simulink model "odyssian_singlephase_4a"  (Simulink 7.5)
settings: Solver=ode23t  StartTime=0.0  StopTime=6  RelTol=1e-6
undefined symbols (not defined in the file or in its folder): dfilt, DiscIntNeverNeededParam
libraries: powerlib x80, powerlib_extras x43, simulink x24, dsparch4 x4
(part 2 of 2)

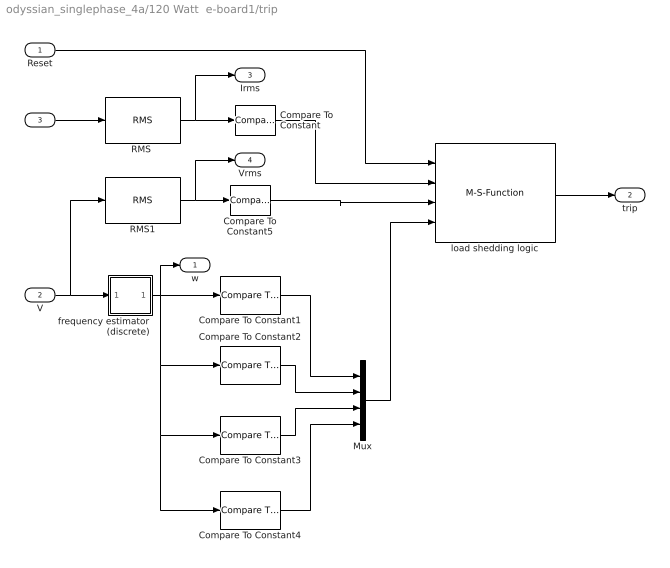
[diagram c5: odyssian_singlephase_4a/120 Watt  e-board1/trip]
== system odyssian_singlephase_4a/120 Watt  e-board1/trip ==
  Reset : Inport
  V : Inport  Port=2
  I : Inport  Port=3
  Compare To Constant : simulink/Logic and Bit Operations/Compare To Constant  SystemSampleTime=-1  relop=>=  const=100  LogicOutDataTypeMode=boolean
  Compare To Constant1 : simulink/Logic and Bit Operations/Compare To Constant  SystemSampleTime=-1  relop=<=  const=59.8  LogicOutDataTypeMode=boolean
  Compare To Constant2 : simulink/Logic and Bit Operations/Compare To Constant  SystemSampleTime=-1  relop=<=  const=59.5  LogicOutDataTypeMode=boolean
  Compare To Constant3 : simulink/Logic and Bit Operations/Compare To Constant  SystemSampleTime=-1  relop=>=  const=60.1  LogicOutDataTypeMode=boolean
  Compare To Constant4 : simulink/Logic and Bit Operations/Compare To Constant  SystemSampleTime=-1  relop=<=  const=58.6  LogicOutDataTypeMode=boolean
  Compare To Constant5 : simulink/Logic and Bit Operations/Compare To Constant  SystemSampleTime=-1  relop=<=  const=100  LogicOutDataTypeMode=boolean
  Mux : Mux
  "RMS " : powerlib_extras/Measurements/RMS  DialogController=POWERSYS.PowerSysDialog  SystemSampleTime=-1  f1=60
  RMS1 : powerlib_extras/Measurements/RMS  DialogController=POWERSYS.PowerSysDialog  SystemSampleTime=-1  f1=60
  frequency estimator (discrete) : Subsystem  mask{dt=0.010}
      mask prompts: dt "sample time"
  load shedding logic : M-S-Function  FunctionName=load_shedding_logic  Parameters=p
  w : Outport  OutDataType=fixdt(1, 16)  OutScaling=2^0
  trip : Outport  Port=2
  Irms : Outport  Port=3  OutDataType=fixdt(1, 16)  OutScaling=2^0
  Vrms : Outport  Port=4  OutDataType=fixdt(1, 16)  OutScaling=2^0
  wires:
  "RMS "/1 -> Compare To Constant/1, Irms/1
  I/1 -> "RMS "/1
  Reset/1 -> load shedding logic/1
  Compare To Constant/1 -> load shedding logic/2
  load shedding logic/1 -> trip/1
  V/1 -> frequency estimator (discrete)/1(v), RMS1/1
  frequency estimator (discrete)/1(w) -> Compare To Constant1/1, w/1, Compare To Constant2/1, Compare To Constant3/1, Compare To Constant4/1
  Compare To Constant1/1 -> Mux/1
  Compare To Constant2/1 -> Mux/2
  Compare To Constant3/1 -> Mux/3
  Compare To Constant4/1 -> Mux/4
  RMS1/1 -> Compare To Constant5/1, Vrms/1
  Compare To Constant5/1 -> load shedding logic/3
  Mux/1 -> load shedding logic/4

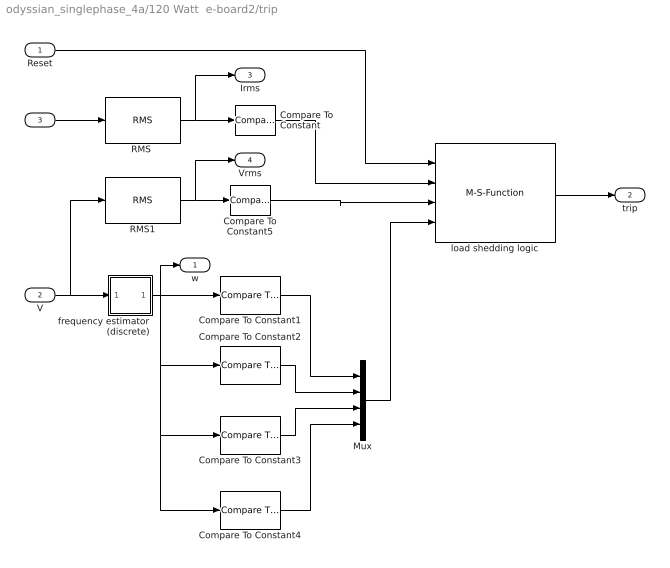
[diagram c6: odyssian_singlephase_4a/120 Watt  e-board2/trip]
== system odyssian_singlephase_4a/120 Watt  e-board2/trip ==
  Reset : Inport
  V : Inport  Port=2
  I : Inport  Port=3
  Compare To Constant : simulink/Logic and Bit Operations/Compare To Constant  SystemSampleTime=-1  relop=>=  const=100  LogicOutDataTypeMode=boolean
  Compare To Constant1 : simulink/Logic and Bit Operations/Compare To Constant  SystemSampleTime=-1  relop=<=  const=59.8  LogicOutDataTypeMode=boolean
  Compare To Constant2 : simulink/Logic and Bit Operations/Compare To Constant  SystemSampleTime=-1  relop=<=  const=59.5  LogicOutDataTypeMode=boolean
  Compare To Constant3 : simulink/Logic and Bit Operations/Compare To Constant  SystemSampleTime=-1  relop=>=  const=60.1  LogicOutDataTypeMode=boolean
  Compare To Constant4 : simulink/Logic and Bit Operations/Compare To Constant  SystemSampleTime=-1  relop=<=  const=58.6  LogicOutDataTypeMode=boolean
  Compare To Constant5 : simulink/Logic and Bit Operations/Compare To Constant  SystemSampleTime=-1  relop=<=  const=100  LogicOutDataTypeMode=boolean
  Mux : Mux
  "RMS " : powerlib_extras/Measurements/RMS  DialogController=POWERSYS.PowerSysDialog  SystemSampleTime=-1  f1=60
  RMS1 : powerlib_extras/Measurements/RMS  DialogController=POWERSYS.PowerSysDialog  SystemSampleTime=-1  f1=60
  frequency estimator (discrete) : Subsystem  mask{dt=0.010}
      mask prompts: dt "sample time"
  load shedding logic : M-S-Function  FunctionName=load_shedding_logic  Parameters=p
  w : Outport  OutDataType=fixdt(1, 16)  OutScaling=2^0
  trip : Outport  Port=2
  Irms : Outport  Port=3  OutDataType=fixdt(1, 16)  OutScaling=2^0
  Vrms : Outport  Port=4  OutDataType=fixdt(1, 16)  OutScaling=2^0
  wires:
  "RMS "/1 -> Compare To Constant/1, Irms/1
  I/1 -> "RMS "/1
  Reset/1 -> load shedding logic/1
  Compare To Constant/1 -> load shedding logic/2
  load shedding logic/1 -> trip/1
  V/1 -> frequency estimator (discrete)/1(v), RMS1/1
  frequency estimator (discrete)/1(w) -> Compare To Constant1/1, w/1, Compare To Constant2/1, Compare To Constant3/1, Compare To Constant4/1
  Compare To Constant1/1 -> Mux/1
  Compare To Constant2/1 -> Mux/2
  Compare To Constant3/1 -> Mux/3
  Compare To Constant4/1 -> Mux/4
  RMS1/1 -> Compare To Constant5/1, Vrms/1
  Compare To Constant5/1 -> load shedding logic/3
  Mux/1 -> load shedding logic/4

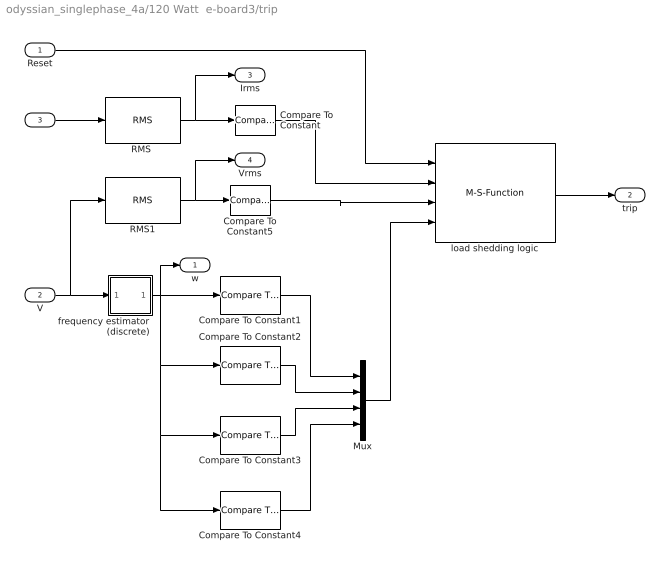
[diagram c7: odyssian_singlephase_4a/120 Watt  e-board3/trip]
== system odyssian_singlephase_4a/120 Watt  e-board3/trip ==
  Reset : Inport
  V : Inport  Port=2
  I : Inport  Port=3
  Compare To Constant : simulink/Logic and Bit Operations/Compare To Constant  SystemSampleTime=-1  relop=>=  const=100  LogicOutDataTypeMode=boolean
  Compare To Constant1 : simulink/Logic and Bit Operations/Compare To Constant  SystemSampleTime=-1  relop=<=  const=59.8  LogicOutDataTypeMode=boolean
  Compare To Constant2 : simulink/Logic and Bit Operations/Compare To Constant  SystemSampleTime=-1  relop=<=  const=59.5  LogicOutDataTypeMode=boolean
  Compare To Constant3 : simulink/Logic and Bit Operations/Compare To Constant  SystemSampleTime=-1  relop=>=  const=60.1  LogicOutDataTypeMode=boolean
  Compare To Constant4 : simulink/Logic and Bit Operations/Compare To Constant  SystemSampleTime=-1  relop=<=  const=58.6  LogicOutDataTypeMode=boolean
  Compare To Constant5 : simulink/Logic and Bit Operations/Compare To Constant  SystemSampleTime=-1  relop=<=  const=100  LogicOutDataTypeMode=boolean
  Mux : Mux
  "RMS " : powerlib_extras/Measurements/RMS  DialogController=POWERSYS.PowerSysDialog  SystemSampleTime=-1  f1=60
  RMS1 : powerlib_extras/Measurements/RMS  DialogController=POWERSYS.PowerSysDialog  SystemSampleTime=-1  f1=60
  frequency estimator (discrete) : Subsystem  mask{dt=0.010}
      mask prompts: dt "sample time"
  load shedding logic : M-S-Function  FunctionName=load_shedding_logic  Parameters=p
  w : Outport  OutDataType=fixdt(1, 16)  OutScaling=2^0
  trip : Outport  Port=2
  Irms : Outport  Port=3  OutDataType=fixdt(1, 16)  OutScaling=2^0
  Vrms : Outport  Port=4  OutDataType=fixdt(1, 16)  OutScaling=2^0
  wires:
  "RMS "/1 -> Compare To Constant/1, Irms/1
  I/1 -> "RMS "/1
  Reset/1 -> load shedding logic/1
  Compare To Constant/1 -> load shedding logic/2
  load shedding logic/1 -> trip/1
  V/1 -> frequency estimator (discrete)/1(v), RMS1/1
  frequency estimator (discrete)/1(w) -> Compare To Constant1/1, w/1, Compare To Constant2/1, Compare To Constant3/1, Compare To Constant4/1
  Compare To Constant1/1 -> Mux/1
  Compare To Constant2/1 -> Mux/2
  Compare To Constant3/1 -> Mux/3
  Compare To Constant4/1 -> Mux/4
  RMS1/1 -> Compare To Constant5/1, Vrms/1
  Compare To Constant5/1 -> load shedding logic/3
  Mux/1 -> load shedding logic/4

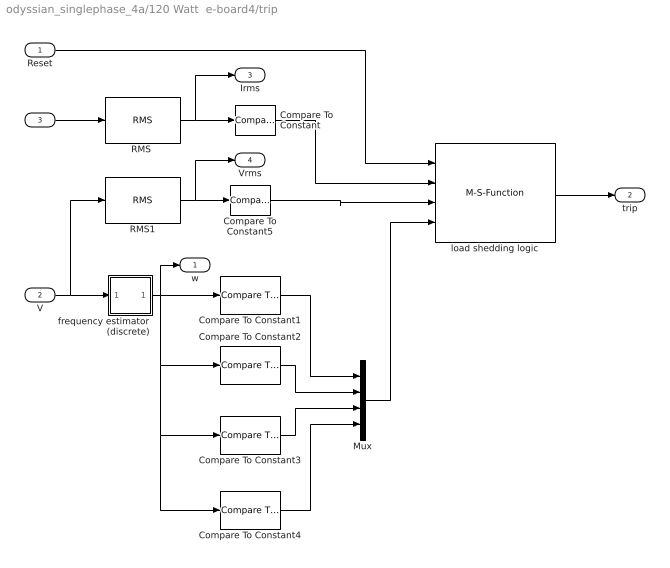
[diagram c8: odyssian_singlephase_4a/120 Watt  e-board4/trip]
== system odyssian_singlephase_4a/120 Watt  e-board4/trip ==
  Reset : Inport
  V : Inport  Port=2
  I : Inport  Port=3
  Compare To Constant : simulink/Logic and Bit Operations/Compare To Constant  SystemSampleTime=-1  relop=>=  const=100  LogicOutDataTypeMode=boolean
  Compare To Constant1 : simulink/Logic and Bit Operations/Compare To Constant  SystemSampleTime=-1  relop=<=  const=59.8  LogicOutDataTypeMode=boolean
  Compare To Constant2 : simulink/Logic and Bit Operations/Compare To Constant  SystemSampleTime=-1  relop=<=  const=59.5  LogicOutDataTypeMode=boolean
  Compare To Constant3 : simulink/Logic and Bit Operations/Compare To Constant  SystemSampleTime=-1  relop=>=  const=60.1  LogicOutDataTypeMode=boolean
  Compare To Constant4 : simulink/Logic and Bit Operations/Compare To Constant  SystemSampleTime=-1  relop=<=  const=58.6  LogicOutDataTypeMode=boolean
  Compare To Constant5 : simulink/Logic and Bit Operations/Compare To Constant  SystemSampleTime=-1  relop=<=  const=100  LogicOutDataTypeMode=boolean
  Mux : Mux
  "RMS " : powerlib_extras/Measurements/RMS  DialogController=POWERSYS.PowerSysDialog  SystemSampleTime=-1  f1=60
  RMS1 : powerlib_extras/Measurements/RMS  DialogController=POWERSYS.PowerSysDialog  SystemSampleTime=-1  f1=60
  frequency estimator (discrete) : Subsystem  mask{dt=0.010}
      mask prompts: dt "sample time"
  load shedding logic : M-S-Function  FunctionName=load_shedding_logic  Parameters=p
  w : Outport  OutDataType=fixdt(1, 16)  OutScaling=2^0
  trip : Outport  Port=2
  Irms : Outport  Port=3  OutDataType=fixdt(1, 16)  OutScaling=2^0
  Vrms : Outport  Port=4  OutDataType=fixdt(1, 16)  OutScaling=2^0
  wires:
  "RMS "/1 -> Compare To Constant/1, Irms/1
  I/1 -> "RMS "/1
  Reset/1 -> load shedding logic/1
  Compare To Constant/1 -> load shedding logic/2
  load shedding logic/1 -> trip/1
  V/1 -> frequency estimator (discrete)/1(v), RMS1/1
  frequency estimator (discrete)/1(w) -> Compare To Constant1/1, w/1, Compare To Constant2/1, Compare To Constant3/1, Compare To Constant4/1
  Compare To Constant1/1 -> Mux/1
  Compare To Constant2/1 -> Mux/2
  Compare To Constant3/1 -> Mux/3
  Compare To Constant4/1 -> Mux/4
  RMS1/1 -> Compare To Constant5/1, Vrms/1
  Compare To Constant5/1 -> load shedding logic/3
  Mux/1 -> load shedding logic/4

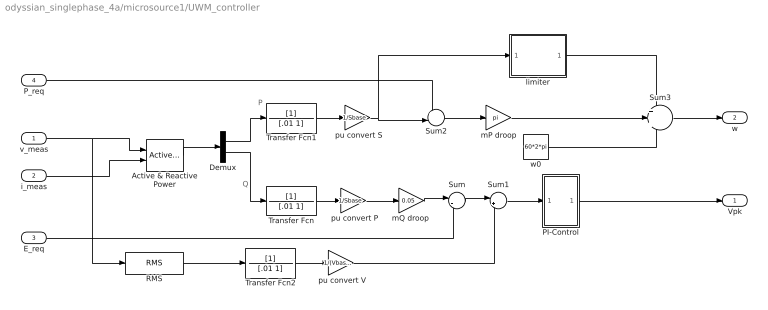
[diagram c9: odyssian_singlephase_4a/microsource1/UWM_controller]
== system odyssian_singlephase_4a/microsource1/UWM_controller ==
  note: P
  note: Q
  v_meas : Inport
  i_meas : Inport  Port=2
  E_req : Inport  Port=3
  P_req : Inport  Port=4
  " pu convert P" : Gain  Gain=1/Sbase  ParameterDataType=sfix(16)  ParameterScaling=2^0  OutDataType=sfix(16)  OutScaling=2^0
  " pu convert S" : Gain  Gain=1/Sbase  ParameterDataType=sfix(16)  ParameterScaling=2^0  OutDataType=sfix(16)  OutScaling=2^0
  " pu convert V" : Gain  Gain=1/(Vbase/sqrt(2))  ParameterDataType=sfix(16)  ParameterScaling=2^0  OutDataType=sfix(16)  OutScaling=2^0
  Active & Reactive Power : powerlib_extras/Measurements/Active & Reactive Power  DialogController=POWERSYS.PowerSysDialog  SystemSampleTime=-1  f1=60
  Demux : Demux  Outputs=2
  PI-Control : Subsystem
  RMS : powerlib_extras/Measurements/RMS  DialogController=POWERSYS.PowerSysDialog  SystemSampleTime=-1  f1=60
  Sum : Sum  Inputs=|-+  OutDataType=sfix(16)  OutScaling=2^0
  Sum1 : Sum  Inputs=|+-  OutDataType=sfix(16)  OutScaling=2^0
  Sum2 : Sum  Inputs=+-|  OutDataType=sfix(16)  OutScaling=2^0
  Sum3 : Sum  Inputs=+++  OutDataType=sfix(16)  OutScaling=2^0
  Transfer Fcn : TransferFcn  Denominator=[.01 1]
  Transfer Fcn1 : TransferFcn  Denominator=[.01 1]
  Transfer Fcn2 : TransferFcn  Denominator=[.01 1]
  limiter : Subsystem
  mP droop : Gain  Gain=pi  ParameterDataType=sfix(16)  ParameterScaling=2^0  OutDataType=sfix(16)  OutScaling=2^0
  "mQ droop " : Gain  Gain=0.05  ParameterDataType=sfix(16)  ParameterScaling=2^0  OutDataType=sfix(16)  OutScaling=2^0
  w0 : Constant  Value=60*2*pi  OutDataType=fixdt(1, 16)  OutScaling=2^0
  Vpk : Outport
  w : Outport  Port=2
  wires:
  Transfer Fcn2/1 -> " pu convert V"/1
  Transfer Fcn/1 -> " pu convert P"/1
  " pu convert P"/1 -> "mQ droop "/1
  Transfer Fcn1/1 -> " pu convert S"/1
  " pu convert S"/1 -> limiter/1(In1), Sum2/2
  i_meas/1 -> Active & Reactive Power/2
  P_req/1 -> Sum2/1
  mP droop/1 -> Sum3/2
  limiter/1(Out1) -> Sum3/1
  w0/1 -> Sum3/3
  Sum2/1 -> mP droop/1
  Sum1/1 -> PI-Control/1(In1)
  Sum/1 -> Sum1/1
  "mQ droop "/1 -> Sum/1
  Demux/2 -> Transfer Fcn/1
  Demux/1 -> Transfer Fcn1/1
  Active & Reactive Power/1 -> Demux/1
  v_meas/1 -> RMS/1, Active & Reactive Power/1
  PI-Control/1(Out1) -> Vpk/1
  Sum3/1 -> w/1
  E_req/1 -> Sum/2
  " pu convert V"/1 -> Sum1/2
  RMS/1 -> Transfer Fcn2/1

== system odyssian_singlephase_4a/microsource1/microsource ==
  Vpk : Inport  OutDataType=fixdt(1, 16)  OutScaling=2^0
  w : Inport  Port=2  OutDataType=fixdt(1, 16)  OutScaling=2^0
  Integrator : Integrator
  Product : Product  OutDataType=sfix(16)  OutScaling=2^0
  phaseA : powerlib/Electrical Sources/Controlled Voltage Source  DialogController=POWERSYS.PowerSysDialog  SystemSampleTime=-1  Initialize=on  Source_Type=AC  Amplitude=0  Phase=0  Frequency=0  Measurements=None
  v_A : Fcn  Expr=cos(u)
  Va : PMIOPort  Tag=PMCPort  Port=1  Side=Right
  Neutral : PMIOPort  Tag=PMCPort  Port=2  Side=Right
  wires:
  Product/1 -> phaseA/1
  Vpk/1 -> Product/1
  w/1 -> Integrator/1
  Integrator/1 -> v_A/1
  v_A/1 -> Product/2
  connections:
  phaseA/RConn1 -- Va/RConn1
  phaseA/LConn1 -- Neutral/RConn1

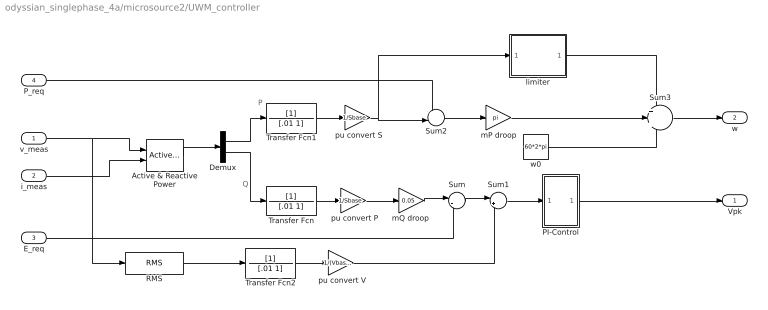
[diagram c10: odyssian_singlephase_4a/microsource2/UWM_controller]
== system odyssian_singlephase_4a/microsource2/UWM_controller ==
  note: P
  note: Q
  v_meas : Inport
  i_meas : Inport  Port=2
  E_req : Inport  Port=3
  P_req : Inport  Port=4
  " pu convert P" : Gain  Gain=1/Sbase  ParameterDataType=sfix(16)  ParameterScaling=2^0  OutDataType=sfix(16)  OutScaling=2^0
  " pu convert S" : Gain  Gain=1/Sbase  ParameterDataType=sfix(16)  ParameterScaling=2^0  OutDataType=sfix(16)  OutScaling=2^0
  " pu convert V" : Gain  Gain=1/(Vbase/sqrt(2))  ParameterDataType=sfix(16)  ParameterScaling=2^0  OutDataType=sfix(16)  OutScaling=2^0
  Active & Reactive Power : powerlib_extras/Measurements/Active & Reactive Power  DialogController=POWERSYS.PowerSysDialog  SystemSampleTime=-1  f1=60
  Demux : Demux  Outputs=2
  PI-Control : Subsystem
  RMS : powerlib_extras/Measurements/RMS  DialogController=POWERSYS.PowerSysDialog  SystemSampleTime=-1  f1=60
  Sum : Sum  Inputs=|-+  OutDataType=sfix(16)  OutScaling=2^0
  Sum1 : Sum  Inputs=|+-  OutDataType=sfix(16)  OutScaling=2^0
  Sum2 : Sum  Inputs=+-|  OutDataType=sfix(16)  OutScaling=2^0
  Sum3 : Sum  Inputs=+++  OutDataType=sfix(16)  OutScaling=2^0
  Transfer Fcn : TransferFcn  Denominator=[.01 1]
  Transfer Fcn1 : TransferFcn  Denominator=[.01 1]
  Transfer Fcn2 : TransferFcn  Denominator=[.01 1]
  limiter : Subsystem
  mP droop : Gain  Gain=pi  ParameterDataType=sfix(16)  ParameterScaling=2^0  OutDataType=sfix(16)  OutScaling=2^0
  "mQ droop " : Gain  Gain=0.05  ParameterDataType=sfix(16)  ParameterScaling=2^0  OutDataType=sfix(16)  OutScaling=2^0
  w0 : Constant  Value=60*2*pi  OutDataType=fixdt(1, 16)  OutScaling=2^0
  Vpk : Outport
  w : Outport  Port=2
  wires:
  Transfer Fcn2/1 -> " pu convert V"/1
  Transfer Fcn/1 -> " pu convert P"/1
  " pu convert P"/1 -> "mQ droop "/1
  Transfer Fcn1/1 -> " pu convert S"/1
  " pu convert S"/1 -> limiter/1(In1), Sum2/2
  i_meas/1 -> Active & Reactive Power/2
  P_req/1 -> Sum2/1
  mP droop/1 -> Sum3/2
  limiter/1(Out1) -> Sum3/1
  w0/1 -> Sum3/3
  Sum2/1 -> mP droop/1
  Sum1/1 -> PI-Control/1(In1)
  Sum/1 -> Sum1/1
  "mQ droop "/1 -> Sum/1
  Demux/2 -> Transfer Fcn/1
  Demux/1 -> Transfer Fcn1/1
  Active & Reactive Power/1 -> Demux/1
  v_meas/1 -> RMS/1, Active & Reactive Power/1
  PI-Control/1(Out1) -> Vpk/1
  Sum3/1 -> w/1
  E_req/1 -> Sum/2
  " pu convert V"/1 -> Sum1/2
  RMS/1 -> Transfer Fcn2/1

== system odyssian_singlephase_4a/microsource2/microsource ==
  Vpk : Inport  OutDataType=fixdt(1, 16)  OutScaling=2^0
  w : Inport  Port=2  OutDataType=fixdt(1, 16)  OutScaling=2^0
  Integrator : Integrator
  Product : Product  OutDataType=sfix(16)  OutScaling=2^0
  phaseA : powerlib/Electrical Sources/Controlled Voltage Source  DialogController=POWERSYS.PowerSysDialog  SystemSampleTime=-1  Initialize=on  Source_Type=AC  Amplitude=0  Phase=0  Frequency=0  Measurements=None
  v_A : Fcn  Expr=cos(u)
  Va : PMIOPort  Tag=PMCPort  Port=1  Side=Right
  Neutral : PMIOPort  Tag=PMCPort  Port=2  Side=Right
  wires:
  Product/1 -> phaseA/1
  Vpk/1 -> Product/1
  w/1 -> Integrator/1
  Integrator/1 -> v_A/1
  v_A/1 -> Product/2
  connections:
  phaseA/RConn1 -- Va/RConn1
  phaseA/LConn1 -- Neutral/RConn1

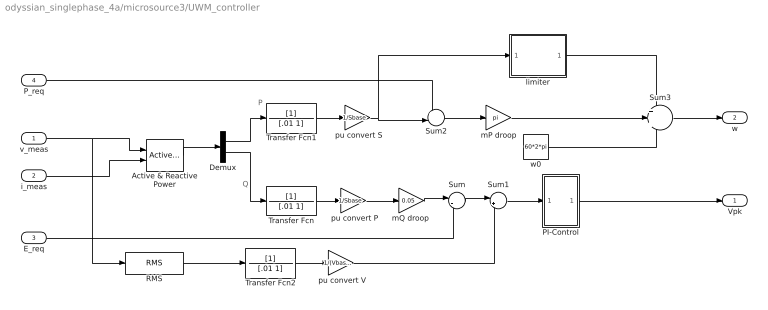
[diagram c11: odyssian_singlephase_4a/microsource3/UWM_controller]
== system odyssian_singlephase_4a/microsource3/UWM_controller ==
  note: P
  note: Q
  v_meas : Inport
  i_meas : Inport  Port=2
  E_req : Inport  Port=3
  P_req : Inport  Port=4
  " pu convert P" : Gain  Gain=1/Sbase  ParameterDataType=sfix(16)  ParameterScaling=2^0  OutDataType=sfix(16)  OutScaling=2^0
  " pu convert S" : Gain  Gain=1/Sbase  ParameterDataType=sfix(16)  ParameterScaling=2^0  OutDataType=sfix(16)  OutScaling=2^0
  " pu convert V" : Gain  Gain=1/(Vbase/sqrt(2))  ParameterDataType=sfix(16)  ParameterScaling=2^0  OutDataType=sfix(16)  OutScaling=2^0
  Active & Reactive Power : powerlib_extras/Measurements/Active & Reactive Power  DialogController=POWERSYS.PowerSysDialog  SystemSampleTime=-1  f1=60
  Demux : Demux  Outputs=2
  PI-Control : Subsystem
  RMS : powerlib_extras/Measurements/RMS  DialogController=POWERSYS.PowerSysDialog  SystemSampleTime=-1  f1=60
  Sum : Sum  Inputs=|-+  OutDataType=sfix(16)  OutScaling=2^0
  Sum1 : Sum  Inputs=|+-  OutDataType=sfix(16)  OutScaling=2^0
  Sum2 : Sum  Inputs=+-|  OutDataType=sfix(16)  OutScaling=2^0
  Sum3 : Sum  Inputs=+++  OutDataType=sfix(16)  OutScaling=2^0
  Transfer Fcn : TransferFcn  Denominator=[.01 1]
  Transfer Fcn1 : TransferFcn  Denominator=[.01 1]
  Transfer Fcn2 : TransferFcn  Denominator=[.01 1]
  limiter : Subsystem
  mP droop : Gain  Gain=pi  ParameterDataType=sfix(16)  ParameterScaling=2^0  OutDataType=sfix(16)  OutScaling=2^0
  "mQ droop " : Gain  Gain=0.05  ParameterDataType=sfix(16)  ParameterScaling=2^0  OutDataType=sfix(16)  OutScaling=2^0
  w0 : Constant  Value=60*2*pi  OutDataType=fixdt(1, 16)  OutScaling=2^0
  Vpk : Outport
  w : Outport  Port=2
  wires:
  Transfer Fcn2/1 -> " pu convert V"/1
  Transfer Fcn/1 -> " pu convert P"/1
  " pu convert P"/1 -> "mQ droop "/1
  Transfer Fcn1/1 -> " pu convert S"/1
  " pu convert S"/1 -> limiter/1(In1), Sum2/2
  i_meas/1 -> Active & Reactive Power/2
  P_req/1 -> Sum2/1
  mP droop/1 -> Sum3/2
  limiter/1(Out1) -> Sum3/1
  w0/1 -> Sum3/3
  Sum2/1 -> mP droop/1
  Sum1/1 -> PI-Control/1(In1)
  Sum/1 -> Sum1/1
  "mQ droop "/1 -> Sum/1
  Demux/2 -> Transfer Fcn/1
  Demux/1 -> Transfer Fcn1/1
  Active & Reactive Power/1 -> Demux/1
  v_meas/1 -> RMS/1, Active & Reactive Power/1
  PI-Control/1(Out1) -> Vpk/1
  Sum3/1 -> w/1
  E_req/1 -> Sum/2
  " pu convert V"/1 -> Sum1/2
  RMS/1 -> Transfer Fcn2/1

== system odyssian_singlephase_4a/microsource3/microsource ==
  Vpk : Inport  OutDataType=fixdt(1, 16)  OutScaling=2^0
  w : Inport  Port=2  OutDataType=fixdt(1, 16)  OutScaling=2^0
  Integrator : Integrator
  Product : Product  OutDataType=sfix(16)  OutScaling=2^0
  phaseA : powerlib/Electrical Sources/Controlled Voltage Source  DialogController=POWERSYS.PowerSysDialog  SystemSampleTime=-1  Initialize=on  Source_Type=AC  Amplitude=0  Phase=0  Frequency=0  Measurements=None
  v_A : Fcn  Expr=cos(u)
  Va : PMIOPort  Tag=PMCPort  Port=1  Side=Right
  Neutral : PMIOPort  Tag=PMCPort  Port=2  Side=Right
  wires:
  Product/1 -> phaseA/1
  Vpk/1 -> Product/1
  w/1 -> Integrator/1
  Integrator/1 -> v_A/1
  v_A/1 -> Product/2
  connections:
  phaseA/RConn1 -- Va/RConn1
  phaseA/LConn1 -- Neutral/RConn1

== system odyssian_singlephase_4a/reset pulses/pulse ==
  Step : Step  Time=tstart  SampleTime=0
  Step1 : Step  Time=tstart+dt  After=-1  SampleTime=0
  Sum : Sum  Inputs=|++  OutDataType=fixdt(1, 16)  OutScaling=2^0
  Out1 : Outport
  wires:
  Step/1 -> Sum/2
  Step1/1 -> Sum/1
  Sum/1 -> Out1/1

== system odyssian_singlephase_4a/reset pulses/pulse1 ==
  Step : Step  Time=tstart  SampleTime=0
  Step1 : Step  Time=tstart+dt  After=-1  SampleTime=0
  Sum : Sum  Inputs=|++  OutDataType=fixdt(1, 16)  OutScaling=2^0
  Out1 : Outport
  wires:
  Step/1 -> Sum/2
  Step1/1 -> Sum/1
  Sum/1 -> Out1/1

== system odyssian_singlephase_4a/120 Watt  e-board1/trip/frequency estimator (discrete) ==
  v : Inport
  Constant : Constant  Value=60  OutDataType=fixdt(1, 16)  OutScaling=2^0
  Fcn : Fcn  Expr=sin(2*pi*u[1])
  Filter Quantized : Subsystem  Tag=BlockMethodSubSystem
  Gain : Gain  Gain=1/150  ParameterDataType=fixdt(1, 16)  ParameterScaling=2^0  OutDataType=fixdt(1, 16)  OutScaling=2^0  SampleTime=dt
  Product : Product  OutDataType=fixdt(1, 16)  OutScaling=2^0
  Scope : Scope
  Sum : Sum  Inputs=|++  OutDataType=fixdt(1, 16)  OutScaling=2^0
  modulo discrete integrator : Subsystem  mask{dt=dt}
      mask prompts: dt "sample time"
  w : Outport  OutDataType=fixdt(1, 16)  OutScaling=2^0
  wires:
  Fcn/1 -> Product/2
  Constant/1 -> Sum/2
  modulo discrete integrator/1(Out1) -> Fcn/1
  Sum/1 -> modulo discrete integrator/1(In1), w/1
  Product/1 -> Filter Quantized/1(In)
  Filter Quantized/1(Out) -> Scope/1, Sum/1
  v/1 -> Gain/1
  Gain/1 -> Product/1

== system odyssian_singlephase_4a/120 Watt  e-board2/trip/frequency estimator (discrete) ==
  v : Inport
  Constant : Constant  Value=60  OutDataType=fixdt(1, 16)  OutScaling=2^0
  Fcn : Fcn  Expr=sin(2*pi*u[1])
  Filter Quantized : Subsystem  Tag=BlockMethodSubSystem
  Gain : Gain  Gain=1/150  ParameterDataType=fixdt(1, 16)  ParameterScaling=2^0  OutDataType=fixdt(1, 16)  OutScaling=2^0  SampleTime=dt
  Product : Product  OutDataType=fixdt(1, 16)  OutScaling=2^0
  Scope : Scope
  Sum : Sum  Inputs=|++  OutDataType=fixdt(1, 16)  OutScaling=2^0
  modulo discrete integrator : Subsystem  mask{dt=dt}
      mask prompts: dt "sample time"
  w : Outport  OutDataType=fixdt(1, 16)  OutScaling=2^0
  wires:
  Fcn/1 -> Product/2
  Constant/1 -> Sum/2
  modulo discrete integrator/1(Out1) -> Fcn/1
  Sum/1 -> modulo discrete integrator/1(In1), w/1
  Product/1 -> Filter Quantized/1(In)
  Filter Quantized/1(Out) -> Scope/1, Sum/1
  v/1 -> Gain/1
  Gain/1 -> Product/1

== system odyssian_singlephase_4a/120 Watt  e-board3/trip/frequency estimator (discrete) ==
  v : Inport
  Constant : Constant  Value=60  OutDataType=fixdt(1, 16)  OutScaling=2^0
  Fcn : Fcn  Expr=sin(2*pi*u[1])
  Filter Quantized : Subsystem  Tag=BlockMethodSubSystem
  Gain : Gain  Gain=1/150  ParameterDataType=fixdt(1, 16)  ParameterScaling=2^0  OutDataType=fixdt(1, 16)  OutScaling=2^0  SampleTime=dt
  Product : Product  OutDataType=fixdt(1, 16)  OutScaling=2^0
  Scope : Scope
  Sum : Sum  Inputs=|++  OutDataType=fixdt(1, 16)  OutScaling=2^0
  modulo discrete integrator : Subsystem  mask{dt=dt}
      mask prompts: dt "sample time"
  w : Outport  OutDataType=fixdt(1, 16)  OutScaling=2^0
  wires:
  Fcn/1 -> Product/2
  Constant/1 -> Sum/2
  modulo discrete integrator/1(Out1) -> Fcn/1
  Sum/1 -> modulo discrete integrator/1(In1), w/1
  Product/1 -> Filter Quantized/1(In)
  Filter Quantized/1(Out) -> Scope/1, Sum/1
  v/1 -> Gain/1
  Gain/1 -> Product/1

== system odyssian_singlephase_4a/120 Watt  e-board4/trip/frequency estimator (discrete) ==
  v : Inport
  Constant : Constant  Value=60  OutDataType=fixdt(1, 16)  OutScaling=2^0
  Fcn : Fcn  Expr=sin(2*pi*u[1])
  Filter Quantized : Subsystem  Tag=BlockMethodSubSystem
  Gain : Gain  Gain=1/150  ParameterDataType=fixdt(1, 16)  ParameterScaling=2^0  OutDataType=fixdt(1, 16)  OutScaling=2^0  SampleTime=dt
  Product : Product  OutDataType=fixdt(1, 16)  OutScaling=2^0
  Scope : Scope
  Sum : Sum  Inputs=|++  OutDataType=fixdt(1, 16)  OutScaling=2^0
  modulo discrete integrator : Subsystem  mask{dt=dt}
      mask prompts: dt "sample time"
  w : Outport  OutDataType=fixdt(1, 16)  OutScaling=2^0
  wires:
  Fcn/1 -> Product/2
  Constant/1 -> Sum/2
  modulo discrete integrator/1(Out1) -> Fcn/1
  Sum/1 -> modulo discrete integrator/1(In1), w/1
  Product/1 -> Filter Quantized/1(In)
  Filter Quantized/1(Out) -> Scope/1, Sum/1
  v/1 -> Gain/1
  Gain/1 -> Product/1

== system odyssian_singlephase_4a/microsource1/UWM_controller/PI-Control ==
  In1 : Inport
  Gain : Gain  Gain=.01  ParameterDataType=sfix(16)  ParameterScaling=2^0  OutDataType=sfix(16)  OutScaling=2^0
  Gain1 : Gain  Gain=5  ParameterDataType=sfix(16)  ParameterScaling=2^0  OutDataType=sfix(16)  OutScaling=2^0
  Gain2 : Gain  Gain=750  ParameterDataType=sfix(16)  ParameterScaling=2^0  OutDataType=sfix(16)  OutScaling=2^0
  Integrator1 : Integrator  LimitOutput=on  UpperSaturationLimit=100  LowerSaturationLimit=-100  ZeroCross=off
  Sum4 : Sum  Inputs=|++  OutDataType=sfix(16)  OutScaling=2^0
  Out1 : Outport
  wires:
  Gain/1 -> Sum4/1
  Integrator1/1 -> Sum4/2
  In1/1 -> Gain1/1, Gain/1
  Gain1/1 -> Integrator1/1
  Sum4/1 -> Gain2/1
  Gain2/1 -> Out1/1

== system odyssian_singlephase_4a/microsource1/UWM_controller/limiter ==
  In1 : Inport
  Discrete-Time Integrator : DiscreteIntegrator  OutDataType=fixdt(1, 16)  OutScaling=2^0  LimitOutput=on  UpperSaturationLimit=0  LowerSaturationLimit=-pi  ICPrevOutput=DiscIntNeverNeededParam  ICPrevScaledInput=DiscIntNeverNeededParam
  Discrete-Time Integrator1 : DiscreteIntegrator  OutDataType=fixdt(1, 16)  OutScaling=2^0  LimitOutput=on  UpperSaturationLimit=pi  LowerSaturationLimit=0  ICPrevOutput=DiscIntNeverNeededParam  ICPrevScaledInput=DiscIntNeverNeededParam
  Kilim : Gain  Gain=30  ParameterDataType=sfix(16)  ParameterScaling=2^0  OutDataType=sfix(16)  OutScaling=2^0
  Kilim1 : Gain  Gain=30  ParameterDataType=sfix(16)  ParameterScaling=2^0  OutDataType=sfix(16)  OutScaling=2^0
  Kplim : Gain  Gain=3  ParameterDataType=sfix(16)  ParameterScaling=2^0  OutDataType=sfix(16)  OutScaling=2^0
  Kplim1 : Gain  Gain=3  ParameterDataType=sfix(16)  ParameterScaling=2^0  OutDataType=sfix(16)  OutScaling=2^0
  Plimit : Constant  Value=1.0  OutDataType=sfix(16)  OutScaling=2^0
  Plimit1 : Constant  Value=0.0  OutDataType=sfix(16)  OutScaling=2^0
  Saturation1 : Saturate  UpperLimit=pi  LowerLimit=0  OutDataType=fixdt(1, 16)  OutScaling=2^0
  Saturation2 : Saturate  UpperLimit=0  LowerLimit=-pi  OutDataType=fixdt(1, 16)  OutScaling=2^0
  Sum1 : Sum  Inputs=-+|  OutDataType=sfix(16)  OutScaling=2^0
  Sum2 : Sum  Inputs=|++  OutDataType=sfix(16)  OutScaling=2^0
  Sum3 : Sum  OutDataType=sfix(16)  OutScaling=2^0
  Sum4 : Sum  Inputs=|+-  OutDataType=sfix(16)  OutScaling=2^0
  Sum9 : Sum  Inputs=|++  OutDataType=sfix(16)  OutScaling=2^0
  Out1 : Outport
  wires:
  Sum3/1 -> Out1/1
  Plimit1/1 -> Sum1/2
  Discrete-Time Integrator1/1 -> Sum2/2
  Kilim1/1 -> Discrete-Time Integrator1/1
  Sum1/1 -> Kilim1/1, Kplim1/1
  In1/1 -> Sum1/1, Sum4/2
  Discrete-Time Integrator/1 -> Sum9/2
  Kilim/1 -> Discrete-Time Integrator/1
  Sum4/1 -> Kilim/1, Kplim/1
  Plimit/1 -> Sum4/1
  Kplim1/1 -> Saturation1/1
  Saturation1/1 -> Sum2/1
  Kplim/1 -> Saturation2/1
  Saturation2/1 -> Sum9/1
  Sum9/1 -> Sum3/1
  Sum2/1 -> Sum3/2

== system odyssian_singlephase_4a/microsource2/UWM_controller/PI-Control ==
  In1 : Inport
  Gain : Gain  Gain=.01  ParameterDataType=sfix(16)  ParameterScaling=2^0  OutDataType=sfix(16)  OutScaling=2^0
  Gain1 : Gain  Gain=5  ParameterDataType=sfix(16)  ParameterScaling=2^0  OutDataType=sfix(16)  OutScaling=2^0
  Gain2 : Gain  Gain=750  ParameterDataType=sfix(16)  ParameterScaling=2^0  OutDataType=sfix(16)  OutScaling=2^0
  Integrator1 : Integrator  LimitOutput=on  UpperSaturationLimit=100  LowerSaturationLimit=-100  ZeroCross=off
  Sum4 : Sum  Inputs=|++  OutDataType=sfix(16)  OutScaling=2^0
  Out1 : Outport
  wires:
  Gain/1 -> Sum4/1
  Integrator1/1 -> Sum4/2
  In1/1 -> Gain1/1, Gain/1
  Gain1/1 -> Integrator1/1
  Sum4/1 -> Gain2/1
  Gain2/1 -> Out1/1

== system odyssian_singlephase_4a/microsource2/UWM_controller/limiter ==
  In1 : Inport
  Discrete-Time Integrator : DiscreteIntegrator  OutDataType=fixdt(1, 16)  OutScaling=2^0  LimitOutput=on  UpperSaturationLimit=0  LowerSaturationLimit=-pi  ICPrevOutput=DiscIntNeverNeededParam  ICPrevScaledInput=DiscIntNeverNeededParam
  Discrete-Time Integrator1 : DiscreteIntegrator  OutDataType=fixdt(1, 16)  OutScaling=2^0  LimitOutput=on  UpperSaturationLimit=pi  LowerSaturationLimit=0  ICPrevOutput=DiscIntNeverNeededParam  ICPrevScaledInput=DiscIntNeverNeededParam
  Kilim : Gain  Gain=30  ParameterDataType=sfix(16)  ParameterScaling=2^0  OutDataType=sfix(16)  OutScaling=2^0
  Kilim1 : Gain  Gain=30  ParameterDataType=sfix(16)  ParameterScaling=2^0  OutDataType=sfix(16)  OutScaling=2^0
  Kplim : Gain  Gain=3  ParameterDataType=sfix(16)  ParameterScaling=2^0  OutDataType=sfix(16)  OutScaling=2^0
  Kplim1 : Gain  Gain=3  ParameterDataType=sfix(16)  ParameterScaling=2^0  OutDataType=sfix(16)  OutScaling=2^0
  Plimit : Constant  Value=1.0  OutDataType=sfix(16)  OutScaling=2^0
  Plimit1 : Constant  Value=0.0  OutDataType=sfix(16)  OutScaling=2^0
  Saturation1 : Saturate  UpperLimit=pi  LowerLimit=0  OutDataType=fixdt(1, 16)  OutScaling=2^0
  Saturation2 : Saturate  UpperLimit=0  LowerLimit=-pi  OutDataType=fixdt(1, 16)  OutScaling=2^0
  Sum1 : Sum  Inputs=-+|  OutDataType=sfix(16)  OutScaling=2^0
  Sum2 : Sum  Inputs=|++  OutDataType=sfix(16)  OutScaling=2^0
  Sum3 : Sum  OutDataType=sfix(16)  OutScaling=2^0
  Sum4 : Sum  Inputs=|+-  OutDataType=sfix(16)  OutScaling=2^0
  Sum9 : Sum  Inputs=|++  OutDataType=sfix(16)  OutScaling=2^0
  Out1 : Outport
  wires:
  Sum3/1 -> Out1/1
  Plimit1/1 -> Sum1/2
  Discrete-Time Integrator1/1 -> Sum2/2
  Kilim1/1 -> Discrete-Time Integrator1/1
  Sum1/1 -> Kilim1/1, Kplim1/1
  In1/1 -> Sum1/1, Sum4/2
  Discrete-Time Integrator/1 -> Sum9/2
  Kilim/1 -> Discrete-Time Integrator/1
  Sum4/1 -> Kilim/1, Kplim/1
  Plimit/1 -> Sum4/1
  Kplim1/1 -> Saturation1/1
  Saturation1/1 -> Sum2/1
  Kplim/1 -> Saturation2/1
  Saturation2/1 -> Sum9/1
  Sum9/1 -> Sum3/1
  Sum2/1 -> Sum3/2

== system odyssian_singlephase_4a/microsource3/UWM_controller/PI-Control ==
  In1 : Inport
  Gain : Gain  Gain=.01  ParameterDataType=sfix(16)  ParameterScaling=2^0  OutDataType=sfix(16)  OutScaling=2^0
  Gain1 : Gain  Gain=5  ParameterDataType=sfix(16)  ParameterScaling=2^0  OutDataType=sfix(16)  OutScaling=2^0
  Gain2 : Gain  Gain=750  ParameterDataType=sfix(16)  ParameterScaling=2^0  OutDataType=sfix(16)  OutScaling=2^0
  Integrator1 : Integrator  LimitOutput=on  UpperSaturationLimit=100  LowerSaturationLimit=-100  ZeroCross=off
  Sum4 : Sum  Inputs=|++  OutDataType=sfix(16)  OutScaling=2^0
  Out1 : Outport
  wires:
  Gain/1 -> Sum4/1
  Integrator1/1 -> Sum4/2
  In1/1 -> Gain1/1, Gain/1
  Gain1/1 -> Integrator1/1
  Sum4/1 -> Gain2/1
  Gain2/1 -> Out1/1

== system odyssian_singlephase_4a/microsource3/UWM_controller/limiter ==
  In1 : Inport
  Discrete-Time Integrator : DiscreteIntegrator  OutDataType=fixdt(1, 16)  OutScaling=2^0  LimitOutput=on  UpperSaturationLimit=0  LowerSaturationLimit=-pi  ICPrevOutput=DiscIntNeverNeededParam  ICPrevScaledInput=DiscIntNeverNeededParam
  Discrete-Time Integrator1 : DiscreteIntegrator  OutDataType=fixdt(1, 16)  OutScaling=2^0  LimitOutput=on  UpperSaturationLimit=pi  LowerSaturationLimit=0  ICPrevOutput=DiscIntNeverNeededParam  ICPrevScaledInput=DiscIntNeverNeededParam
  Kilim : Gain  Gain=30  ParameterDataType=sfix(16)  ParameterScaling=2^0  OutDataType=sfix(16)  OutScaling=2^0
  Kilim1 : Gain  Gain=30  ParameterDataType=sfix(16)  ParameterScaling=2^0  OutDataType=sfix(16)  OutScaling=2^0
  Kplim : Gain  Gain=3  ParameterDataType=sfix(16)  ParameterScaling=2^0  OutDataType=sfix(16)  OutScaling=2^0
  Kplim1 : Gain  Gain=3  ParameterDataType=sfix(16)  ParameterScaling=2^0  OutDataType=sfix(16)  OutScaling=2^0
  Plimit : Constant  Value=1.0  OutDataType=sfix(16)  OutScaling=2^0
  Plimit1 : Constant  Value=0.0  OutDataType=sfix(16)  OutScaling=2^0
  Saturation1 : Saturate  UpperLimit=pi  LowerLimit=0  OutDataType=fixdt(1, 16)  OutScaling=2^0
  Saturation2 : Saturate  UpperLimit=0  LowerLimit=-pi  OutDataType=fixdt(1, 16)  OutScaling=2^0
  Sum1 : Sum  Inputs=-+|  OutDataType=sfix(16)  OutScaling=2^0
  Sum2 : Sum  Inputs=|++  OutDataType=sfix(16)  OutScaling=2^0
  Sum3 : Sum  OutDataType=sfix(16)  OutScaling=2^0
  Sum4 : Sum  Inputs=|+-  OutDataType=sfix(16)  OutScaling=2^0
  Sum9 : Sum  Inputs=|++  OutDataType=sfix(16)  OutScaling=2^0
  Out1 : Outport
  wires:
  Sum3/1 -> Out1/1
  Plimit1/1 -> Sum1/2
  Discrete-Time Integrator1/1 -> Sum2/2
  Kilim1/1 -> Discrete-Time Integrator1/1
  Sum1/1 -> Kilim1/1, Kplim1/1
  In1/1 -> Sum1/1, Sum4/2
  Discrete-Time Integrator/1 -> Sum9/2
  Kilim/1 -> Discrete-Time Integrator/1
  Sum4/1 -> Kilim/1, Kplim/1
  Plimit/1 -> Sum4/1
  Kplim1/1 -> Saturation1/1
  Saturation1/1 -> Sum2/1
  Kplim/1 -> Saturation2/1
  Saturation2/1 -> Sum9/1
  Sum9/1 -> Sum3/1
  Sum2/1 -> Sum3/2

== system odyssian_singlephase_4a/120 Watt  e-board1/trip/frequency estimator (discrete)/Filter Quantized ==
  In : Inport
  Input Quantizer : DataTypeConversion  OutDataTypeMode=Specify via dialog  OutDataType=fixdt(1,16,15)  OutDataTypeStr=fixdt(1,16,15)  RndMeth=Round
  filter : dsparch4/Biquad Filter  DialogController=dspdialog.BiquadFilter  DialogControllerArgs=DataTag0  IIRFiltStruct=Direct form II  CoeffSource=Specify via dialog  BiQuadCoeffs=[1 -1.35890654546667 1 1 -1.77683423091592 0.868775728611993;1 1 0 1 -0.84680556917748 0]  a0Flag=Warning  IC=0  ICnum=0  ICden=0  firstCoeffMode=Binary point scaling  firstCoeffWordLength=16  firstCoeffFracLength=14  outputMode=Binary point scaling  outputWordLength=16  outputFracLength=11  accumMode=Binary point scaling  accumWordLength=40  accumFracLength=29  denAccumFracLength=29  prodOutputMode=Binary point scaling  prodOutputWordLength=32  prodOutputFracLength=29  denProdOutputFracLength=29  memoryMode=Binary point scaling  memoryWordLength=16  memoryFracLength=15  secondMemoryFracLength=15  roundingMode=Convergent  overflowMode=off  ScaleValues=[0.0483208011510974;0.227336456672284;1]  optimizeScaleValues=on  ScaleValueMode=Specify via input port (g)  scaleValueFracLength=17  stageInputMode=Binary point scaling  stageOutputMode=Binary point scaling  stageInputWordLength=16  stageInputFracLength=12  stageOutputWordLength=16  stageOutputFracLength=11  FilterSource=Specify via dialog  dfiltObjectName=dfilt.df2tsos([1 0.3 0.4],[1 0.1 0.2])
  Out : Outport
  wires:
  In/1 -> Input Quantizer/1
  Input Quantizer/1 -> filter/1
  filter/1 -> Out/1

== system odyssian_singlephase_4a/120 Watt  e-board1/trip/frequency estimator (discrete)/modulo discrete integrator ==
  In1 : Inport
  Abs : Abs
  Constant1 : Constant  OutDataType=sfix(16)  OutScaling=2^0
  Discrete-Time Integrator : DiscreteIntegrator  ExternalReset=rising  InitialConditionSource=external  SampleTime=dt  OutDataType=fixdt(1, 16)  OutScaling=2^0  UpperSaturationLimit=100  LowerSaturationLimit=-100  ShowStatePort=on  ICPrevOutput=DiscIntNeverNeededParam  ICPrevScaledInput=DiscIntNeverNeededParam
  Gain1 : Gain  Gain=1+.0001  ParameterDataType=sfix(16)  ParameterScaling=2^0  OutDataType=sfix(16)  OutScaling=2^0
  IC : InitialCondition  Value=0
  Math Function : Math  Operator=rem  OutDataType=sfix(16)  OutScaling=2^0
  Relational Operator : RelationalOperator
  Out1 : Outport
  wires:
  Relational Operator/1 -> Discrete-Time Integrator/2
  Discrete-Time Integrator/State -> Gain1/1
  Gain1/1 -> Abs/1
  Constant1/1 -> Relational Operator/2, Math Function/2
  Abs/1 -> Relational Operator/1, Math Function/1
  In1/1 -> Discrete-Time Integrator/1
  Discrete-Time Integrator/1 -> Out1/1
  IC/1 -> Discrete-Time Integrator/3
  Math Function/1 -> IC/1

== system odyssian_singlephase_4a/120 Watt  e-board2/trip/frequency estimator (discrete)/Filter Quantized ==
  In : Inport
  Input Quantizer : DataTypeConversion  OutDataTypeMode=Specify via dialog  OutDataType=fixdt(1,16,15)  OutDataTypeStr=fixdt(1,16,15)  RndMeth=Round
  filter : dsparch4/Biquad Filter  DialogController=dspdialog.BiquadFilter  DialogControllerArgs=DataTag1  IIRFiltStruct=Direct form II  CoeffSource=Specify via dialog  BiQuadCoeffs=[1 -1.35890654546667 1 1 -1.77683423091592 0.868775728611993;1 1 0 1 -0.84680556917748 0]  a0Flag=Warning  IC=0  ICnum=0  ICden=0  firstCoeffMode=Binary point scaling  firstCoeffWordLength=16  firstCoeffFracLength=14  outputMode=Binary point scaling  outputWordLength=16  outputFracLength=11  accumMode=Binary point scaling  accumWordLength=40  accumFracLength=29  denAccumFracLength=29  prodOutputMode=Binary point scaling  prodOutputWordLength=32  prodOutputFracLength=29  denProdOutputFracLength=29  memoryMode=Binary point scaling  memoryWordLength=16  memoryFracLength=15  secondMemoryFracLength=15  roundingMode=Convergent  overflowMode=off  ScaleValues=[0.0483208011510974;0.227336456672284;1]  optimizeScaleValues=on  ScaleValueMode=Specify via input port (g)  scaleValueFracLength=17  stageInputMode=Binary point scaling  stageOutputMode=Binary point scaling  stageInputWordLength=16  stageInputFracLength=12  stageOutputWordLength=16  stageOutputFracLength=11  FilterSource=Specify via dialog  dfiltObjectName=dfilt.df2tsos([1 0.3 0.4],[1 0.1 0.2])
  Out : Outport
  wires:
  In/1 -> Input Quantizer/1
  Input Quantizer/1 -> filter/1
  filter/1 -> Out/1

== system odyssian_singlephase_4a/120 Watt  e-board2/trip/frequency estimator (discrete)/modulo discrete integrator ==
  In1 : Inport
  Abs : Abs
  Constant1 : Constant  OutDataType=sfix(16)  OutScaling=2^0
  Discrete-Time Integrator : DiscreteIntegrator  ExternalReset=rising  InitialConditionSource=external  SampleTime=dt  OutDataType=fixdt(1, 16)  OutScaling=2^0  UpperSaturationLimit=100  LowerSaturationLimit=-100  ShowStatePort=on  ICPrevOutput=DiscIntNeverNeededParam  ICPrevScaledInput=DiscIntNeverNeededParam
  Gain1 : Gain  Gain=1+.0001  ParameterDataType=sfix(16)  ParameterScaling=2^0  OutDataType=sfix(16)  OutScaling=2^0
  IC : InitialCondition  Value=0
  Math Function : Math  Operator=rem  OutDataType=sfix(16)  OutScaling=2^0
  Relational Operator : RelationalOperator
  Out1 : Outport
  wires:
  Relational Operator/1 -> Discrete-Time Integrator/2
  Discrete-Time Integrator/State -> Gain1/1
  Gain1/1 -> Abs/1
  Constant1/1 -> Relational Operator/2, Math Function/2
  Abs/1 -> Relational Operator/1, Math Function/1
  In1/1 -> Discrete-Time Integrator/1
  Discrete-Time Integrator/1 -> Out1/1
  IC/1 -> Discrete-Time Integrator/3
  Math Function/1 -> IC/1

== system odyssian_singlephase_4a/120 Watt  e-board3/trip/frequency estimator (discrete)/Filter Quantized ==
  In : Inport
  Input Quantizer : DataTypeConversion  OutDataTypeMode=Specify via dialog  OutDataType=fixdt(1,16,15)  OutDataTypeStr=fixdt(1,16,15)  RndMeth=Round
  filter : dsparch4/Biquad Filter  DialogController=dspdialog.BiquadFilter  DialogControllerArgs=DataTag2  IIRFiltStruct=Direct form II  CoeffSource=Specify via dialog  BiQuadCoeffs=[1 -1.35890654546667 1 1 -1.77683423091592 0.868775728611993;1 1 0 1 -0.84680556917748 0]  a0Flag=Warning  IC=0  ICnum=0  ICden=0  firstCoeffMode=Binary point scaling  firstCoeffWordLength=16  firstCoeffFracLength=14  outputMode=Binary point scaling  outputWordLength=16  outputFracLength=11  accumMode=Binary point scaling  accumWordLength=40  accumFracLength=29  denAccumFracLength=29  prodOutputMode=Binary point scaling  prodOutputWordLength=32  prodOutputFracLength=29  denProdOutputFracLength=29  memoryMode=Binary point scaling  memoryWordLength=16  memoryFracLength=15  secondMemoryFracLength=15  roundingMode=Convergent  overflowMode=off  ScaleValues=[0.0483208011510974;0.227336456672284;1]  optimizeScaleValues=on  ScaleValueMode=Specify via input port (g)  scaleValueFracLength=17  stageInputMode=Binary point scaling  stageOutputMode=Binary point scaling  stageInputWordLength=16  stageInputFracLength=12  stageOutputWordLength=16  stageOutputFracLength=11  FilterSource=Specify via dialog  dfiltObjectName=dfilt.df2tsos([1 0.3 0.4],[1 0.1 0.2])
  Out : Outport
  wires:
  In/1 -> Input Quantizer/1
  Input Quantizer/1 -> filter/1
  filter/1 -> Out/1

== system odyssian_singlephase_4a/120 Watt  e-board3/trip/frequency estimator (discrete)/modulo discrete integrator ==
  In1 : Inport
  Abs : Abs
  Constant1 : Constant  OutDataType=sfix(16)  OutScaling=2^0
  Discrete-Time Integrator : DiscreteIntegrator  ExternalReset=rising  InitialConditionSource=external  SampleTime=dt  OutDataType=fixdt(1, 16)  OutScaling=2^0  UpperSaturationLimit=100  LowerSaturationLimit=-100  ShowStatePort=on  ICPrevOutput=DiscIntNeverNeededParam  ICPrevScaledInput=DiscIntNeverNeededParam
  Gain1 : Gain  Gain=1+.0001  ParameterDataType=sfix(16)  ParameterScaling=2^0  OutDataType=sfix(16)  OutScaling=2^0
  IC : InitialCondition  Value=0
  Math Function : Math  Operator=rem  OutDataType=sfix(16)  OutScaling=2^0
  Relational Operator : RelationalOperator
  Out1 : Outport
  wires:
  Relational Operator/1 -> Discrete-Time Integrator/2
  Discrete-Time Integrator/State -> Gain1/1
  Gain1/1 -> Abs/1
  Constant1/1 -> Relational Operator/2, Math Function/2
  Abs/1 -> Relational Operator/1, Math Function/1
  In1/1 -> Discrete-Time Integrator/1
  Discrete-Time Integrator/1 -> Out1/1
  IC/1 -> Discrete-Time Integrator/3
  Math Function/1 -> IC/1

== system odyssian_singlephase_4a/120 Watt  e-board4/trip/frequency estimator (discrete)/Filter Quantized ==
  In : Inport
  Input Quantizer : DataTypeConversion  OutDataTypeMode=Specify via dialog  OutDataType=fixdt(1,16,15)  OutDataTypeStr=fixdt(1,16,15)  RndMeth=Round
  filter : dsparch4/Biquad Filter  DialogController=dspdialog.BiquadFilter  DialogControllerArgs=DataTag3  IIRFiltStruct=Direct form II  CoeffSource=Specify via dialog  BiQuadCoeffs=[1 -1.35890654546667 1 1 -1.77683423091592 0.868775728611993;1 1 0 1 -0.84680556917748 0]  a0Flag=Warning  IC=0  ICnum=0  ICden=0  firstCoeffMode=Binary point scaling  firstCoeffWordLength=16  firstCoeffFracLength=14  outputMode=Binary point scaling  outputWordLength=16  outputFracLength=11  accumMode=Binary point scaling  accumWordLength=40  accumFracLength=29  denAccumFracLength=29  prodOutputMode=Binary point scaling  prodOutputWordLength=32  prodOutputFracLength=29  denProdOutputFracLength=29  memoryMode=Binary point scaling  memoryWordLength=16  memoryFracLength=15  secondMemoryFracLength=15  roundingMode=Convergent  overflowMode=off  ScaleValues=[0.0483208011510974;0.227336456672284;1]  optimizeScaleValues=on  ScaleValueMode=Specify via input port (g)  scaleValueFracLength=17  stageInputMode=Binary point scaling  stageOutputMode=Binary point scaling  stageInputWordLength=16  stageInputFracLength=12  stageOutputWordLength=16  stageOutputFracLength=11  FilterSource=Specify via dialog  dfiltObjectName=dfilt.df2tsos([1 0.3 0.4],[1 0.1 0.2])
  Out : Outport
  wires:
  In/1 -> Input Quantizer/1
  Input Quantizer/1 -> filter/1
  filter/1 -> Out/1

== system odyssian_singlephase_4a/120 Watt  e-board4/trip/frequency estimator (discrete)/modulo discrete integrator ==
  In1 : Inport
  Abs : Abs
  Constant1 : Constant  OutDataType=sfix(16)  OutScaling=2^0
  Discrete-Time Integrator : DiscreteIntegrator  ExternalReset=rising  InitialConditionSource=external  SampleTime=dt  OutDataType=fixdt(1, 16)  OutScaling=2^0  UpperSaturationLimit=100  LowerSaturationLimit=-100  ShowStatePort=on  ICPrevOutput=DiscIntNeverNeededParam  ICPrevScaledInput=DiscIntNeverNeededParam
  Gain1 : Gain  Gain=1+.0001  ParameterDataType=sfix(16)  ParameterScaling=2^0  OutDataType=sfix(16)  OutScaling=2^0
  IC : InitialCondition  Value=0
  Math Function : Math  Operator=rem  OutDataType=sfix(16)  OutScaling=2^0
  Relational Operator : RelationalOperator
  Out1 : Outport
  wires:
  Relational Operator/1 -> Discrete-Time Integrator/2
  Discrete-Time Integrator/State -> Gain1/1
  Gain1/1 -> Abs/1
  Constant1/1 -> Relational Operator/2, Math Function/2
  Abs/1 -> Relational Operator/1, Math Function/1
  In1/1 -> Discrete-Time Integrator/1
  Discrete-Time Integrator/1 -> Out1/1
  IC/1 -> Discrete-Time Integrator/3
  Math Function/1 -> IC/1
